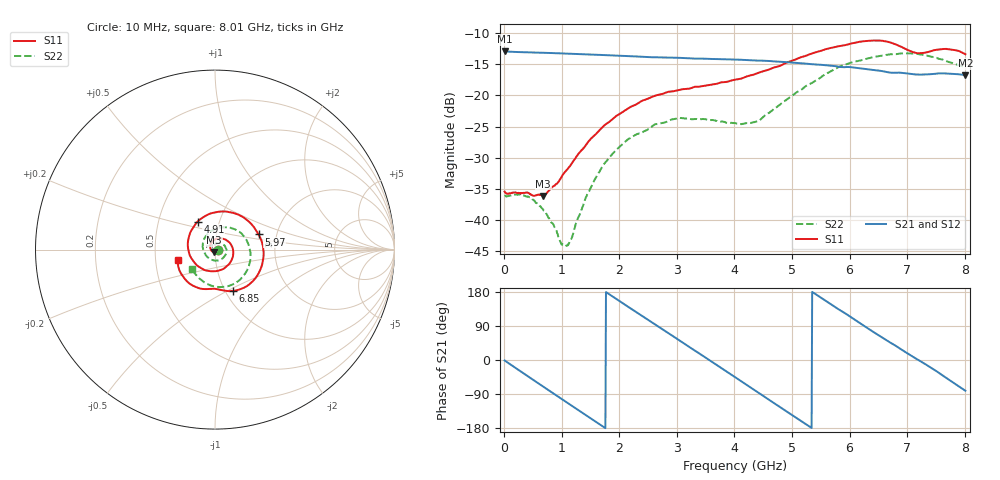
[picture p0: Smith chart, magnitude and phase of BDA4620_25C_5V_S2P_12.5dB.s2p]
!Agilent Technologies,E5071B,MY42404982,A.09.10
!Date: Wed May 06 09:00:47 2026
!Data & Calibration Information:
!Freq	S11:SOLT2(ON)	S21:SOLT2(ON)	S12:SOLT2(ON)	S22:SOLT2(ON)
# Hz S RI R 50
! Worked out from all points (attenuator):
!   801 points, 10 MHz to 8.01 GHz, reference 50 ohm
!   highest |S21| = -12.93 dB at 10 MHz (marker M1); lowest = -16.7 dB at 8.01 GHz (marker M2)
!   lowest |S11| = -36.2 dB at 680 MHz (marker M3), VSWR 1.03, Z = 49.6 - j1.49 ohm
!   |S11| at or under -10 dB: start of sweep to end of sweep
!   |S22| runs from -44.2 to -13.2 dB; largest |S21 - S12| = 0.00097
!   S11 on the Smith chart (normalised r, x): 10 MHz: 1.03, -0.00; 4.91 GHz: 0.79, +0.25; 5.97 GHz: 1.61, +0.29; 6.85 GHz: 1.09, -0.53; 8.01 GHz: 0.65, -0.08
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1e7  0.0168 -0.00122  0.2257 -0.00483  0.2259 -0.0049  0.0155 -0.000707
4.3e8  0.00846 -0.0141  0.1582 -0.1558  0.1583 -0.1562  0.0135 -0.00727
6.8e8  -0.00413 -0.015  0.0748 -0.2071  0.0747 -0.2076  0.00746 -0.00945
1.06e9  -0.0243 0.000795  -0.0705 -0.2055  -0.0707 -0.2057  -0.00474 -0.00391
1.16e9  -0.0262 0.0089  -0.1051 -0.1889  -0.1056 -0.1892  -0.00694 -0.000174
1.35e9  -0.0259 0.0257  -0.1605 -0.1424  -0.1607 -0.1427  -0.00905 0.00818
1.6e9  -0.0126 0.0475  -0.2038 -0.0597  -0.2041 -0.0597  -0.00632 0.0212
1.9e9  0.019 0.0628  -0.2034 0.0504  -0.2038 0.0506  0.00698 0.0338
2.31e9  0.0714 0.0471  -0.1173 0.1688  -0.1174 0.169  0.035 0.0342
2.68e9  0.1012 -0.00338  0.00676 0.2023  0.0069 0.2025  0.0565 0.017
3.4e9  0.031 -0.1134  0.1897 0.0553  0.1901 0.0551  0.0448 -0.0464
4.01e9  -0.1032 -0.0852  0.1369 -0.1378  0.137 -0.1381  -0.0259 -0.054
4.41e9  -0.1508 0.0138  0.0149 -0.1898  0.0147 -0.1904  -0.0615 -0.00928
4.91e9  -0.0972 0.156  -0.1334 -0.128  -0.1337 -0.1283  -0.048 0.0795
5.35e9  0.0463 0.2129  -0.1782 0.00084  -0.1785 0.000875  0.0321 0.1222
5.97e9  0.2426 0.0842  -0.0805 0.1489  -0.0805 0.1491  0.1671 0.0665
6.33e9  0.2653 -0.0729  0.0222 0.1605  0.0223 0.1607  0.1978 -0.022
6.68e9  0.1705 -0.2076  0.1019 0.1141  0.1024 0.1144  0.1778 -0.1174
6.85e9  0.1005 -0.2303  0.1284 0.0821  0.1287 0.0823  0.1492 -0.1563
7.19e9  0.0017 -0.2182  0.147 0.00101  0.1474 0.00115  0.0607 -0.2066
7.54e9  -0.1001 -0.2112  0.1262 -0.0815  0.1264 -0.0814  -0.0366 -0.1946
8.01e9  -0.207 -0.0557  0.0225 -0.1437  0.0227 -0.1441  -0.1262 -0.1096
